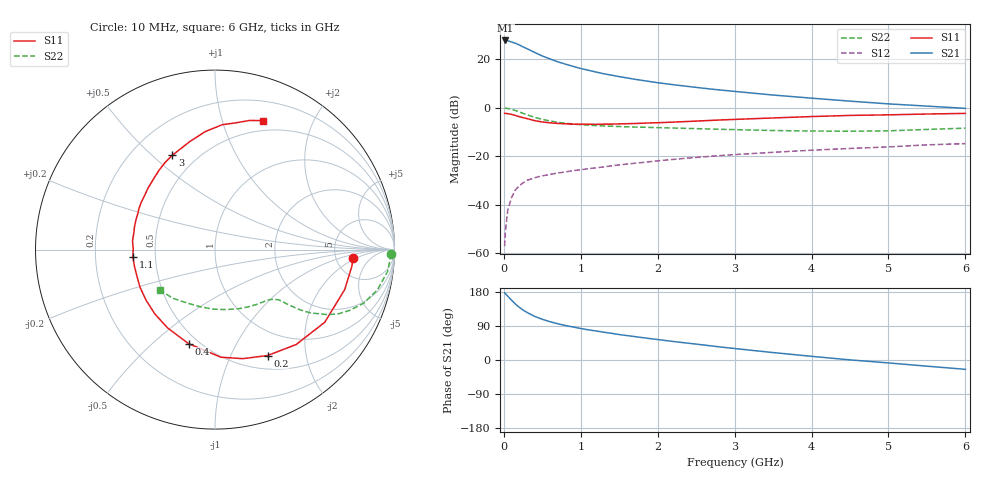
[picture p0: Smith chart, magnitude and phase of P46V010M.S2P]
! SIEMENS Small Signal Semiconductors
! BFP182
! Si NPN RF Bipolar Junction Transistor in SOT143
! VCE = 6 V  IC = 10 mA
! Common Emitter S-Parameters:  March  1996
# GHz  S  MA  R  50
!  f  S11  S21  S12  S22
! GHz  MAG  ANG  MAG  ANG  MAG  ANG  MAG  ANG
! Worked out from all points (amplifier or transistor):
!   36 points, 10 MHz to 6 GHz, reference 50 ohm
!   highest |S21| = 27.8 dB at 20 MHz (marker M1)
!   |S21| within 3 dB of that: start of sweep to 273.5 MHz
!   unconditionally stable (mu >= 1): 1.218 GHz to 5.476 GHz
!   at 250 MHz: K = 0.31, MSG = 28.0 dB, |S12| = -31.0 dB
!   at 1.4 GHz: K = 1.05, MAG = 17.4 dB, |S12| = -23.9 dB
!   at 6 GHz: K = 0.95, MSG = 7.3 dB, |S12| = -14.8 dB
!   lowest NFmin = 1.50 dB at 450 MHz
!   S11 on the Smith chart (normalised r, x): 10 MHz: 7.31, -1.64; 200 MHz: 0.67, -1.39; 400 MHz: 0.44, -0.66; 1.1 GHz: 0.37, -0.04; 3 GHz: 0.37, +0.58; 6 GHz: 0.39, +1.37
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0.01  0.7698 -3.4  24.3 177.3  0.0014 86.5  0.9819 -1.4
0.02  0.7684 -6.9  24.52 175.5  0.0028 85.7  0.9784 -2.8
0.05  0.7563 -17.1  24.17 168.4  0.0076 83.6  0.9694 -7.2
0.1  0.7334 -33.5  22.78 157.9  0.0141 72.7  0.9325 -13.9
0.15  0.6957 -49.5  21.51 147.8  0.0202 65.8  0.881 -19.8
0.2  0.6588 -63.6  19.86 139.2  0.0247 61.2  0.8246 -24.2
0.25  0.6271 -75.7  18.05 131.8  0.0283 57.1  0.7707 -27.8
0.3  0.6004 -86.9  16.62 125.7  0.0319 53.3  0.7194 -30.2
0.4  0.5443 -105.7  13.91 115.1  0.0361 49.3  0.637 -33.6
0.5  0.5103 -121.1  11.72 107.4  0.0395 45.7  0.5777 -35.4
0.6  0.4908 -133.0  10.22 101.1  0.0423 44.9  0.5353 -36.3
0.7  0.4766 -143.6  8.895 95.7  0.0451 44.3  0.5041 -37.0
0.9  0.46 -160.5  7.168 87.1  0.0507 44.3  0.4621 -37.9
1.1  0.4595 -174.9  5.946 79.6  0.0556 44.6  0.4389 -39.3
1.5  0.4658 164.5  4.404 67.1  0.0665 44.5  0.4112 -42.9
1.8  0.481 151.8  3.677 59.1  0.0744 44.1  0.3978 -46.7
2.2  0.507 137.1  3.002 48.9  0.0862 42.3  0.3833 -52.8
3  0.5765 114.4  2.181 30.3  0.1085 37.6  0.3551 -67.9
3.5  0.6178 103.2  1.835 19.6  0.1208 34.0  0.3402 -79.2
4.5  0.6969 86.7  1.373 0.3  0.145 26.6  0.3288 -104.7
5.5  0.7449 75.0  1.085 -16.3  0.1721 19.6  0.3584 -130.8
6  0.7672 69.5  0.975 -24.6  0.1828 15.0  0.3807 -143.4
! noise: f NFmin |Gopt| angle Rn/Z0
0.45  1.5  0.26  43  0.28
0.9  1.6  0.24  87  0.22
1.8  2.1  0.2  170  0.2
